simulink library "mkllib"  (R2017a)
settings: Solver=ode45  StartTime=0.0  StopTime=10.0  RelTol=1e-3  EnableMultiTasking=on
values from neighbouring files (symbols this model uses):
  A = csint_helper(dr,0)    [asxycsJac.m]    (also in dlstc.m = (dzx/drx)^2*rry./(rry + drx/2); fbtopt.m = (1./err (kk)).*A(kk,:))
  a = (d4 - d1) *     0.5    [asxyJac.m]    (also in bslvmex.m = a1 - A*b; fbtxana.m = 0.35)
libraries: mkllib x8

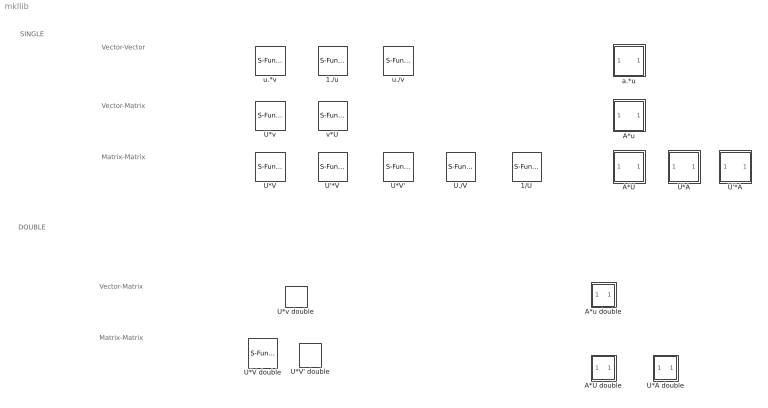
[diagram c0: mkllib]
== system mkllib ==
  note: Vector-Vector
  note: Vector-Matrix
  note: Matrix-Matrix
  note: Matrix-Matrix
  note: Vector-Matrix
  note: DOUBLE
  note: SINGLE
  1./u : S-Function  FunctionName=svinvcsf  SFunctionDeploymentMode=off  EnableBusSupport=off
  1/U : S-Function  FunctionName=sminvcsf  SFunctionDeploymentMode=off  EnableBusSupport=off
  A*U : Subsystem
  A*U double : Subsystem
  A*u : Subsystem
  A*u double : Subsystem
  U'*A : Subsystem
  U'*V : S-Function  FunctionName=smmutvncsf  Parameters=a  SFunctionDeploymentMode=off  EnableBusSupport=off
  U*A : Subsystem
  U*A double : Subsystem
  U*V : S-Function  FunctionName=smmunvncsf  Parameters=a  SFunctionDeploymentMode=off  EnableBusSupport=off
  U*V double : S-Function  FunctionName=dmmunvncsf  Parameters=a  SFunctionDeploymentMode=off  EnableBusSupport=off
  U*V' : S-Function  FunctionName=smmunvtcsf  Parameters=a  SFunctionDeploymentMode=off  EnableBusSupport=off
  U*V' double : S-Function  FunctionName=dmmunvtcsf  Parameters=a  SFunctionDeploymentMode=off  EnableBusSupport=off
  U*v : S-Function  FunctionName=smvunvcsf  Parameters=a  SFunctionDeploymentMode=off  EnableBusSupport=off
  U*v double : S-Function  FunctionName=dmvunvcsf  Parameters=a  SFunctionDeploymentMode=off  EnableBusSupport=off
  U./V : S-Function  FunctionName=smdivuvcsf  SFunctionDeploymentMode=off  EnableBusSupport=off
  a.*u : Subsystem
  u.*v : S-Function  FunctionName=svvuvcsf  SFunctionDeploymentMode=off  EnableBusSupport=off
  u./v : S-Function  FunctionName=svdivuvcsf  SFunctionDeploymentMode=off  EnableBusSupport=off
  v*U : S-Function  FunctionName=smvutvcsf  Parameters=alpha  SFunctionDeploymentMode=off  EnableBusSupport=off

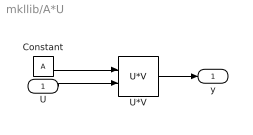
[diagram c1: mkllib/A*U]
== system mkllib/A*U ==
  U : Inport
  Constant : Constant  Value=A  VectorParams1D=off  OutDataTypeStr=single
  U*V : mkllib/U*V  a=1
  y : Outport
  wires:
  U*V/1 -> y/1
  Constant/1 -> U*V/1
  U/1 -> U*V/2

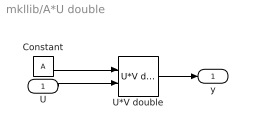
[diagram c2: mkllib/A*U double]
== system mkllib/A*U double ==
  U : Inport
  Constant : Constant  Value=A  VectorParams1D=off  OutDataTypeStr=double
  U*V double : mkllib/U*V double  a=1
  y : Outport
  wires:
  U*V double/1 -> y/1
  Constant/1 -> U*V double/1
  U/1 -> U*V double/2

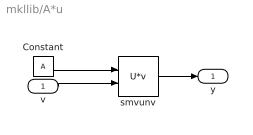
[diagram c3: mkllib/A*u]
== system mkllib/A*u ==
  v : Inport
  Constant : Constant  Value=A  VectorParams1D=off  OutDataTypeStr=single
  smvunv : mkllib/U*v  a=1
  y : Outport
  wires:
  smvunv/1 -> y/1
  Constant/1 -> smvunv/1
  v/1 -> smvunv/2

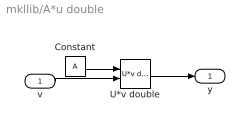
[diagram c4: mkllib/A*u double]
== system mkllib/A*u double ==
  v : Inport
  Constant : Constant  Value=A  VectorParams1D=off  OutDataTypeStr=double
  U*v double : mkllib/U*v double  a=1
  y : Outport
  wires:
  U*v double/1 -> y/1
  Constant/1 -> U*v double/1
  v/1 -> U*v double/2

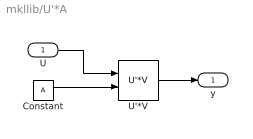
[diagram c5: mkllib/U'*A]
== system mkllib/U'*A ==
  U : Inport
  Constant : Constant  Value=A  VectorParams1D=off  OutDataTypeStr=single
  U'*V : mkllib/U'*V  a=1
  y : Outport
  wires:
  Constant/1 -> U'*V/2
  U/1 -> U'*V/1
  U'*V/1 -> y/1

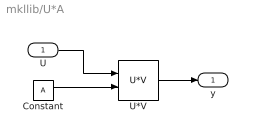
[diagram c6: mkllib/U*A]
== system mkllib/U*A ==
  U : Inport
  Constant : Constant  Value=A  VectorParams1D=off  OutDataTypeStr=single
  U*V : mkllib/U*V  a=1
  y : Outport
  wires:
  U*V/1 -> y/1
  U/1 -> U*V/1
  Constant/1 -> U*V/2

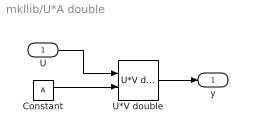
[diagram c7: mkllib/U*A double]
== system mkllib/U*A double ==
  U : Inport
  Constant : Constant  Value=A  VectorParams1D=off  OutDataTypeStr=Inherit: Inherit via back propagation
  U*V double : mkllib/U*V double  a=1
  y : Outport
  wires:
  U*V double/1 -> y/1
  U/1 -> U*V double/1
  Constant/1 -> U*V double/2

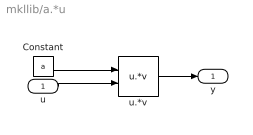
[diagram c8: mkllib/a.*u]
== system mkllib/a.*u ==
  u : Inport
  Constant : Constant  Value=a  OutDataTypeStr=single
  u.*v : mkllib/u.*v
  y : Outport
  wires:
  u/1 -> u.*v/2
  Constant/1 -> u.*v/1
  u.*v/1 -> y/1
